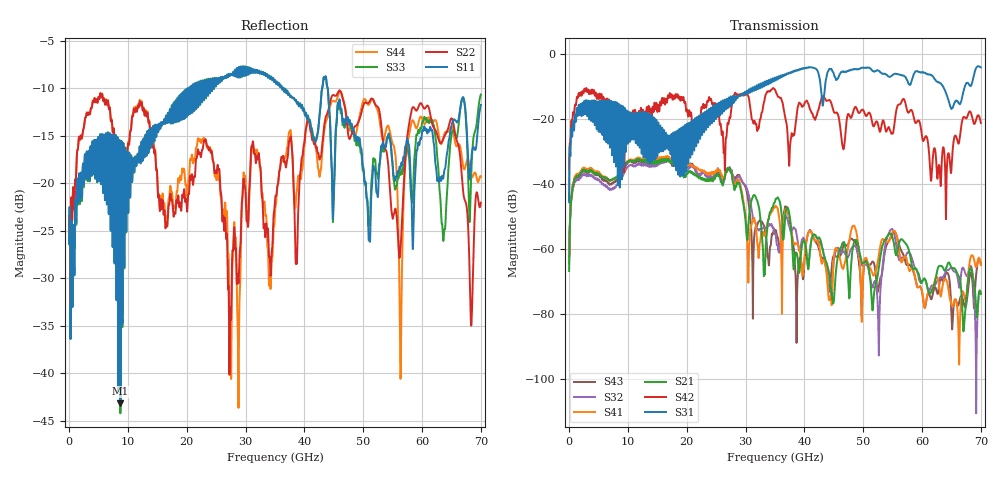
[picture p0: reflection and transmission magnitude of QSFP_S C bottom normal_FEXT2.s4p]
! AWR Design Environment (8415) Tue Jan 08 12:46:14 2019
! Document = 'QSFP Channel_S'
! nPorts: 4, nXvals: 7001
# HZ S DB R 50
!Freq DBS11 AngS11 DBS12 AngS12 DBS13 AngS13 DBS14 AngS14
!	DBS21 AngS21 DBS22 AngS22 DBS23 AngS23 DBS24 AngS24
!	DBS31 AngS31 DBS32 AngS32 DBS33 AngS33 DBS34 AngS34
!	DBS41 AngS41 DBS42 AngS42 DBS43 AngS43 DBS44 AngS44
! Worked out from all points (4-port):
!   7000 points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, 10 MHz to 70 GHz, reference 50 ohm
!   strongest paths, dB at 10 MHz, 17.51 GHz, 35.01 GHz, 52.51 GHz, 70 GHz:
!     S31: -45.6, -27.8, -7.4, -5.0, -4.0
!     S42: -45.1, -12.8, -10.9, -21.6, -21.2
!     S21: -66.8, -33.7, -45.3, -67.5, -73.8
!     S41: -64.5, -32.9, -46.9, -63.5, -64.9
!     S32: -62.3, -33.6, -55.4, -79.6, -73.8
!     S43: -62.2, -34.4, -54.8, -73.1, -64.8
!   lowest |S11| = -43.2 dB at 8.73 GHz (marker M1), VSWR 1.01, Z = 49.5 - j0.488 ohm
!   |S11| at or under -10 dB: start of sweep to 20.43 GHz; 36.44 GHz to 43.04 GHz (6.602 GHz wide, 16.6 % of centre); 43.96 GHz to end of sweep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
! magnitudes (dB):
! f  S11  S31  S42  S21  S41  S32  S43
! 10 MHz  -26.4  -45.6  -45.1  -66.8  -64.5  -62.3  -62.2
! 2.62 GHz  -17.8  -14.3  -10.6  -35.8  -35.2  -37.1  -36.1
! 8.73 GHz  -43.2  -17.0  -26.7  -36.2  -36.4  -38.6  -37.2
! 27.26 GHz  -8.7  -15.6  -19.5  -35.1  -35.0  -34.8  -35.1
! 44.38 GHz  -13.7  -4.6  -14.3  -70.3  -74.7  -71.0  -70.8
! 48.33 GHz  -14.3  -4.6  -17.4  -58.7  -52.9  -59.3  -57.3
! 70 GHz  -11.8  -4.0  -21.2  -73.8  -64.9  -73.8  -64.8
